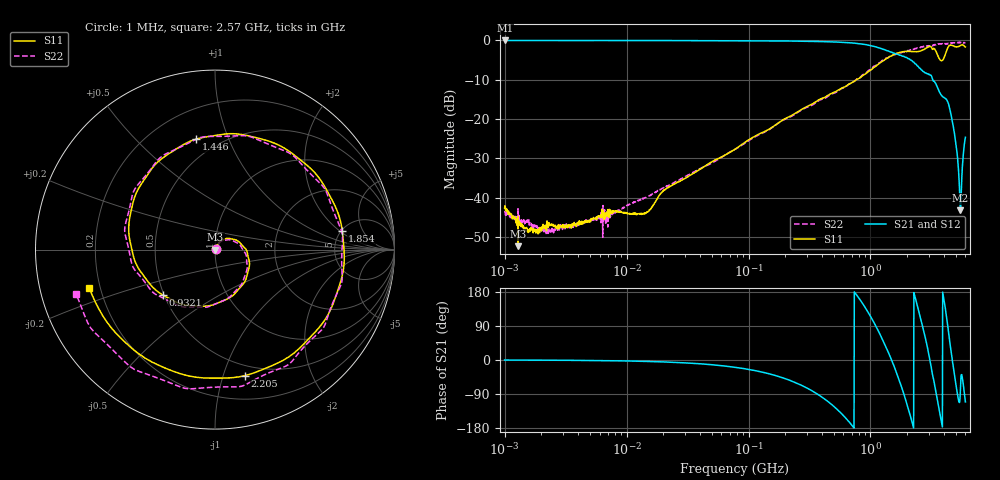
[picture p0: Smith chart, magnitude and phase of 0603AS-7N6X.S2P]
!s-Parameter Generated by FASTRON Sdn. Bhd.
!FASTRON P/N : 0603AS-7N6X
!Keysight Technologies: E5071C_MY46733604_B.14.02
!Date: Mon Dec 04 11:21:04 2023
!Version  :Rev01  Mon Dec 04 11:21:04 2023
!Data & Calibration Information:
!Freq  S11:SOLT2(ON)  S21:SOLT2(ON)  S12:SOLT2(ON)  S22:SOLT2(ON)
!PortZ  Port1:50+j0  Port2:50+j0
!When reading reference impedance value at option line is always used.
! Remarks : This data is being provided solely for informational purposes.
# Hz S dB R 50
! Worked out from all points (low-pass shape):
!   1601 points, 1 MHz to 6 GHz, reference 50 ohm
!   highest |S21| = -0.03 dB at 1.006 MHz (marker M1); lowest = -43.2 dB at 5.468 GHz (marker M2)
!   |S21| within 3 dB of the highest: start of sweep to 1.497 GHz
!   lowest |S11| = -52.3 dB at 1.288 MHz (marker M3), VSWR 1.00, Z = 50.2 + j0.00197 ohm
!   |S11| at or under -10 dB: start of sweep to 766.7 MHz
!   |S22| runs from -50.0 to -0.5 dB; largest |S21 - S12| = 0.006
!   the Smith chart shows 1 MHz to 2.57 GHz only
!   S11 on the Smith chart (normalised r, x): 1 MHz: 1.01, +0.00; 932.1 MHz: 0.49, -0.29; 1.446 GHz: 0.38, +0.77; 1.854 GHz: 5.12, +2.16; 2.205 GHz: 0.40, -1.18; 2.57 GHz: 0.16, -0.15
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1000000  -42.55 18.5  -0.04 -0.1  -0.05 -0.2  -43.35 18.1
1006392  -42.03 18.8  -0.03 -0.1  -0.05 -0.2  -43.58 15.3
1287650  -52.26 0.5  -0.05 -0.2  -0.04 -0.2  -42.77 4.7
4277066  -46.68 38.4  -0.05 -1.1  -0.05 -1.1  -46.43 40.5
1.823719e7  -39.74 61.9  -0.05 -4.6  -0.06 -4.6  -38.07 57.8
7.757876e7  -27.65 61.6  -0.08 -19.3  -0.09 -19.3  -27.66 57.6
3.307917e8  -16.20 8.3  -0.26 -81.1  -0.26 -81.1  -16.47 3.3
6.640706e8  -11.14 -70.8  -0.61 -162.4  -0.60 -162.4  -11.17 -72.7
9.321099e8  -8.28 -139.0  -1.13 131.7  -1.13 131.7  -8.08 -136.6
1.414819e9  -4.28 106.6  -2.78 16.7  -2.78 16.7  -4.25 103.3
1.44567e9  -4.09 99.6  -2.93 9.9  -2.92 9.8  -4.01 96.9
1.854267e9  -2.89 8.2  -4.05 -83.8  -4.06 -83.9  -2.95 3.6
2.205051e9  -2.83 -76.7  -5.32 -167.2  -5.32 -167.2  -2.25 -77.2
2.570242e9  -2.70 -162.9  -7.24 110.1  -7.22 110.2  -1.81 -162.5
3.068351e9  -1.53 94.5  -8.76 0.8  -8.73 0.8  -1.44 82.3
3.462469e9  -2.95 11.7  -11.32 -91.1  -11.31 -91.4  -1.00 -5.2
3.867453e9  -5.12 -69.9  -14.19 -172.8  -14.19 -173.1  -0.84 -99.2
4.231938e9  -2.37 -157.5  -15.22 106.6  -15.23 106.2  -0.85 175.7
4.628987e9  -1.25 107.2  -19.72 11.9  -19.73 11.6  -0.64 89.2
5.048685e9  -1.68 26.4  -26.77 -69.8  -26.79 -70.1  -0.56 -1.2
5.468383e9  -1.32 -61.0  -43.19 -73.3  -43.25 -73.4  -0.62 -93.2
6e9  -1.69 177.3  -24.63 -110.5  -24.63 -110.5  -0.56 161.8
